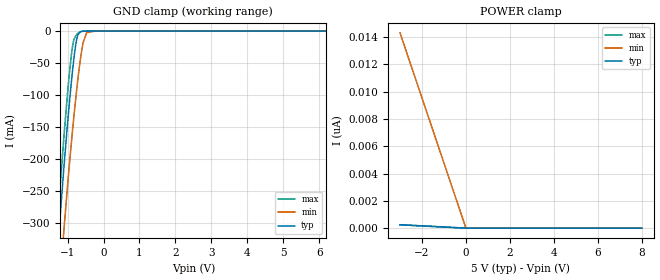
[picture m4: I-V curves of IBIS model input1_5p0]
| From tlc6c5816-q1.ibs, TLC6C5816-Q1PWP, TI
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|   input1_5p0 Model
[Model]   input1_5p0
Model_type   Input
Vinl = 0.7
Vinh = 2.4
|   typ   min   max
C_comp   3.497pF   3.417pF   3.545pF
|  Where Nom  PVT is Nominal Process, 5.0V,  27C
|   Fast PVT is Strong Process,  5.5V, -40C
|   Slow PVT is Weak Process,   4.5V, 150C
[Voltage Range]   5   4.5   5.5
|Junction Temperature
[Temperature Range]   27   150   -40
[Power Clamp Reference]   5   4.5   5.5
[GND Clamp Reference]   0   0   0
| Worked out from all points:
|   GND clamp passes 1 mA (typ) near -0.64 V on its own axis
[GND Clamp]
|   Voltage   I(typ)   I(min)   I(max)
-3V       -1.77A     -1.797A    -1.766A
-1.526V   -539.5mA   -625.1mA   -499.1mA
-1.24V    -313.5mA   -409.1mA   -266.6mA
-1.097V   -208.3mA   -306.3mA   -160.5mA
-976mV    -127.7mA   -224.5mA   -80.96mA
-888mV    -75.4mA    -169.5mA   -33.62mA
-778mV    -22.65mA   -107.3mA   -7.729mA
-657mV    -1.483mA   -49.1mA    -1.437mA
-569mV    -169.5uA   -17.97mA   -200.2uA
-470mV    -12.55uA   -2.508mA   -11.42uA
-239mV    0A         -5.717uA   0A
8V        0A         0A         0A
[POWER Clamp]
|   Voltage   I(typ)   I(min)   I(max)
-3V       247.7pA    14.29nA    247.8pA
0V        0A         0A         0A
8V        0A         0A         0A
